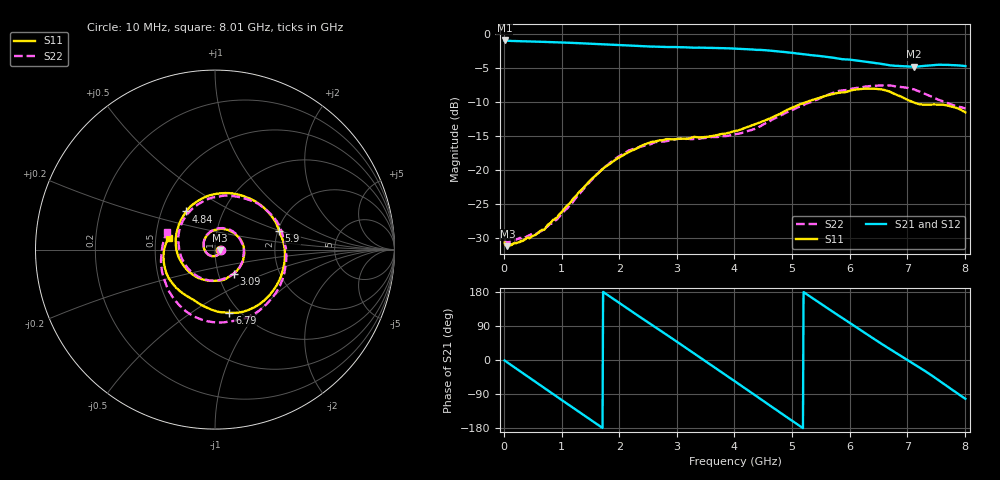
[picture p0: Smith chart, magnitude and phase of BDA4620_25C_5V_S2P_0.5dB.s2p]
!Agilent Technologies,E5071B,MY42404982,A.09.10
!Date: Wed May 06 08:58:10 2026
!Data & Calibration Information:
!Freq	S11:SOLT2(ON)	S21:SOLT2(ON)	S12:SOLT2(ON)	S22:SOLT2(ON)
# Hz S RI R 50
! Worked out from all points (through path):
!   801 points, 10 MHz to 8.01 GHz, reference 50 ohm
!   highest |S21| = -0.95 dB at 10 MHz (marker M1); lowest = -4.8 dB at 7.11 GHz (marker M2)
!   group delay of S21, straight-line fit = 285 ps
!   lowest |S11| = -31.2 dB at 60 MHz (marker M3), VSWR 1.06, Z = 52.8 - j0.44 ohm
!   |S11| at or under -10 dB: start of sweep to 5.248 GHz; 7.097 GHz to end of sweep
!   |S22| runs from -30.7 to -7.5 dB; largest |S21 - S12| = 0.0038
!   S11 on the Smith chart (normalised r, x): 10 MHz: 1.06, -0.00; 3.09 GHz: 1.18, -0.33; 4.84 GHz: 0.67, +0.31; 5.9 GHz: 2.03, +0.50; 6.79 GHz: 0.90, -0.73; 8.01 GHz: 0.59, +0.08
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1e7  0.0292 -0.00209  0.8962 -0.0192  0.8971 -0.0191  0.0307 -0.00194
6e7  0.0273 -0.00416  0.8861 -0.1027  0.8883 -0.1042  0.0291 -0.00323
3.6e8  0.0219 -0.0216  0.6935 -0.547  0.6943 -0.5488  0.0243 -0.0208
7.3e8  -0.00934 -0.037  0.1944 -0.8522  0.1939 -0.8533  -0.00563 -0.0376
1.03e9  -0.0471 -0.0197  -0.2749 -0.8199  -0.2758 -0.8205  -0.0439 -0.0222
1.35e9  -0.064 0.0332  -0.6735 -0.5265  -0.6734 -0.527  -0.0639 0.0292
1.93e9  0.0282 0.1154  -0.7714 0.3125  -0.772 0.3134  0.0222 0.1189
2.32e9  0.1235 0.0774  -0.3794 0.7247  -0.381 0.7253  0.1205 0.084
2.68e9  0.1631 -0.0229  0.1257 0.7963  0.1265 0.7971  0.161 -0.00715
3.09e9  0.104 -0.1345  0.6206 0.5035  0.6226 0.5031  0.1209 -0.119
3.54e9  -0.0264 -0.1739  0.7841 -0.102  0.7851 -0.1034  -0.00541 -0.1731
4.01e9  -0.1619 -0.1055  0.4313 -0.6509  0.4313 -0.6523  -0.149 -0.1069
4.41e9  -0.2187 0.0348  -0.11 -0.7552  -0.1123 -0.757  -0.2024 0.0315
4.84e9  -0.1601 0.2128  -0.5942 -0.4399  -0.5953 -0.4398  -0.1363 0.2172
5.35e9  0.0965 0.3131  -0.67 0.1933  -0.671 0.1941  0.12 0.2951
5.9e9  0.3573 0.1051  -0.2058 0.6191  -0.2054 0.619  0.3769 0.083
6.26e9  0.3712 -0.1396  0.1938 0.5966  0.1959 0.5969  0.3807 -0.1508
6.68e9  0.1534 -0.347  0.5086 0.299  0.5107 0.2995  0.1919 -0.373
6.79e9  0.0798 -0.3522  0.5474 0.2033  0.549 0.2023  0.1143 -0.3953
7.11e9  -0.0861 -0.3025  0.5666 -0.1003  0.5677 -0.1011  -0.1071 -0.377
7.62e9  -0.2637 -0.148  0.284 -0.521  0.2842 -0.5231  -0.2936 -0.1277
8.01e9  -0.257 0.0668  -0.1255 -0.5675  -0.1265 -0.569  -0.2663 0.0979
